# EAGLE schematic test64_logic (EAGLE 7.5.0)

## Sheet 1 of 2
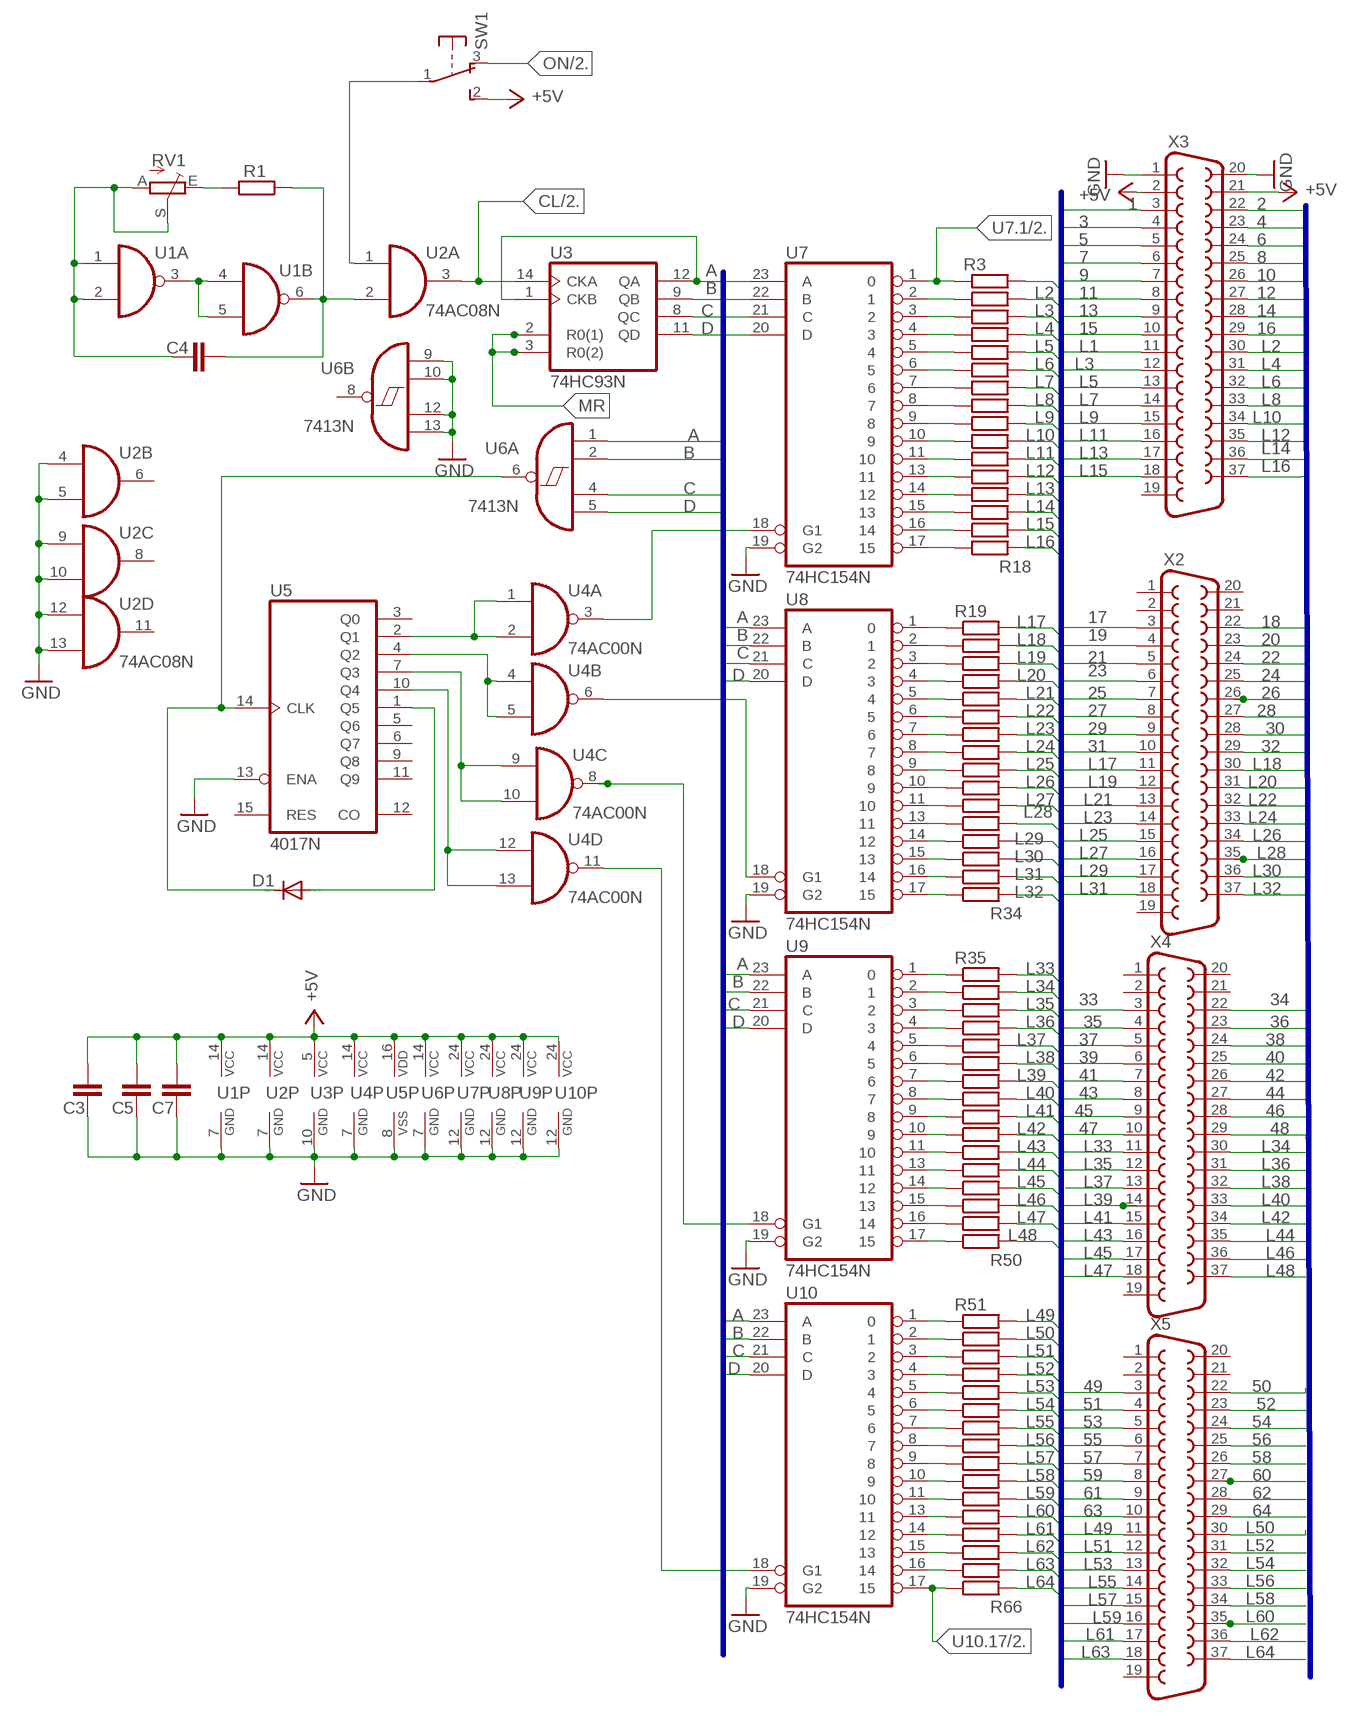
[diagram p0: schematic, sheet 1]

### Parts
C3  C-EUC1206  [C1206]
C4  C-EUC1206  [C1206]
C5  C-EUC1206  [C1206]
C7  C-EUC1206  [C1206]
D1  1N4148DO35-7  [DO35-7]
R1  R-EU_R1206  [R1206]
R3  R-EU_R1206  [R1206]
R4  R-EU_R1206  [R1206]
R5  R-EU_R1206  [R1206]
R6  R-EU_R1206  [R1206]
R7  R-EU_R1206  [R1206]
R8  R-EU_R1206  [R1206]
R9  R-EU_R1206  [R1206]
R10  R-EU_R1206  [R1206]
R11  R-EU_R1206  [R1206]
R12  R-EU_R1206  [R1206]
R13  R-EU_R1206  [R1206]
R14  R-EU_R1206  [R1206]
R15  R-EU_R1206  [R1206]
R16  R-EU_R1206  [R1206]
R17  R-EU_R1206  [R1206]
R18  R-EU_R1206  [R1206]
R19  R-EU_R1206  [R1206]
R20  R-EU_R1206  [R1206]
R21  R-EU_R1206  [R1206]
R22  R-EU_R1206  [R1206]
R23  R-EU_R1206  [R1206]
R24  R-EU_R1206  [R1206]
R25  R-EU_R1206  [R1206]
R26  R-EU_R1206  [R1206]
R27  R-EU_R1206  [R1206]
R28  R-EU_R1206  [R1206]
R29  R-EU_R1206  [R1206]
R30  R-EU_R1206  [R1206]
R31  R-EU_R1206  [R1206]
R32  R-EU_R1206  [R1206]
R33  R-EU_R1206  [R1206]
R34  R-EU_R1206  [R1206]
R35  R-EU_R1206  [R1206]
R36  R-EU_R1206  [R1206]
R37  R-EU_R1206  [R1206]
R38  R-EU_R1206  [R1206]
R39  R-EU_R1206  [R1206]
R40  R-EU_R1206  [R1206]
R41  R-EU_R1206  [R1206]
R42  R-EU_R1206  [R1206]
R43  R-EU_R1206  [R1206]
R44  R-EU_R1206  [R1206]
R45  R-EU_R1206  [R1206]
R46  R-EU_R1206  [R1206]
R47  R-EU_R1206  [R1206]
R48  R-EU_R1206  [R1206]
R49  R-EU_R1206  [R1206]
R50  R-EU_R1206  [R1206]
R51  R-EU_R1206  [R1206]
R52  R-EU_R1206  [R1206]
R53  R-EU_R1206  [R1206]
R54  R-EU_R1206  [R1206]
R55  R-EU_R1206  [R1206]
R56  R-EU_R1206  [R1206]
R57  R-EU_R1206  [R1206]
R58  R-EU_R1206  [R1206]
R59  R-EU_R1206  [R1206]
R60  R-EU_R1206  [R1206]
R61  R-EU_R1206  [R1206]
R62  R-EU_R1206  [R1206]
R63  R-EU_R1206  [R1206]
R64  R-EU_R1206  [R1206]
R65  R-EU_R1206  [R1206]
R66  R-EU_R1206  [R1206]
RV1  TRIM_EU-CT6  [CT6]
SW1  9077-1  [9077-1]
U1  74AC00N  [DIL14]
U2  74AC08N  [DIL14]
U3  74HC93N  [DIL14]
U4  74AC00N  [DIL14]
U5  4017N  [DIL16]
U6  7413N  [DIL14]
U7  74HC154N  [DIL24-6]
U8  74HC154N  [DIL24-6]
U9  74HC154N  [DIL24-6]
U10  74HC154N  [DIL24-6]
X2  F37V  [F37V]
X3  F37V  [F37V]
X4  F37V  [F37V]
X5  F37V  [F37V]

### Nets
1: X3.3 ; also sheet 2
2: X3.22 ; also sheet 2
3: X3.4 ; also sheet 2
4: X3.23 ; also sheet 2
5: X3.5 ; also sheet 2
6: X3.24 ; also sheet 2
7: X3.6 ; also sheet 2
8: X3.25 ; also sheet 2
9: X3.7 ; also sheet 2
10: X3.26 ; also sheet 2
11: X3.8 ; also sheet 2
12: X3.27 ; also sheet 2
13: X3.9 ; also sheet 2
14: X3.28 ; also sheet 2
15: X3.10 ; also sheet 2
16: X3.29 ; also sheet 2
17: X2.3 ; also sheet 2
18: X2.22 ; also sheet 2
19: X2.4 ; also sheet 2
20: X2.23 ; also sheet 2
21: X2.5 ; also sheet 2
22: X2.24 ; also sheet 2
23: X2.6 ; also sheet 2
24: X2.25 ; also sheet 2
25: X2.7 ; also sheet 2
26: X2.26 ; also sheet 2
27: X2.8 ; also sheet 2
28: X2.27 ; also sheet 2
29: X2.9 ; also sheet 2
30: X2.28 ; also sheet 2
31: X2.10 ; also sheet 2
32: X2.29 ; also sheet 2
33: X4.3 ; also sheet 2
34: X4.22 ; also sheet 2
35: X4.4 ; also sheet 2
36: X4.23 ; also sheet 2
37: X4.5 ; also sheet 2
38: X4.24 ; also sheet 2
39: X4.6 ; also sheet 2
40: X4.25 ; also sheet 2
41: X4.7 ; also sheet 2
42: X4.26 ; also sheet 2
43: X4.8 ; also sheet 2
44: X4.27 ; also sheet 2
45: X4.9 ; also sheet 2
46: X4.28 ; also sheet 2
47: X4.10 ; also sheet 2
48: X4.29 ; also sheet 2
49: X5.3 ; also sheet 2
50: X5.22 ; also sheet 2
51: X5.4 ; also sheet 2
52: X5.23 ; also sheet 2
53: X5.5 ; also sheet 2
54: X5.24 ; also sheet 2
55: X5.6 ; also sheet 2
56: X5.25 ; also sheet 2
57: X5.7 ; also sheet 2
58: X5.26 ; also sheet 2
59: X5.8 ; also sheet 2
60: X5.27 ; also sheet 2
61: X5.9 ; also sheet 2
62: X5.28 ; also sheet 2
63: X5.10 ; also sheet 2
64: X5.29 ; also sheet 2
+5V: C3.2 C5.2 C7.2 SW1.2(S) U1.14(P:VCC) U2.14(P:VCC) U3.5(VCC) U4.14(P:VCC) U5.16(VDD) U6.14(P:VCC) U7.24(VCC) U8.24(VCC) U9.24(VCC) U10.24(VCC) X3.2 X3.21 ; also sheet 2
A: U3.1(CKB) U3.12(QA) U6.1(A:I0) U7.23(A) U8.23(A) U9.23(A) U10.23(A)
B: U3.9(QB) U6.2(A:I1) U7.22(B) U8.22(B) U9.22(B) U10.22(B)
C: U3.8(QC) U6.4(A:I2) U7.21(C) U8.21(C) U9.21(C) U10.21(C)
CL: U2.3(A:O) U3.14(CKA) ; also sheet 2
D: U3.11(QD) U6.5(A:I3) U7.20(D) U8.20(D) U9.20(D) U10.20(D)
GND: C3.1 C5.1 C7.1 U1.7(P:GND) U2.4(B:I0) U2.5(B:I1) U2.7(P:GND) U2.9(C:I0) U2.10(C:I1) U2.12(D:I0) U2.13(D:I1) U3.10(GND) U4.7(P:GND) U5.8(VSS) U5.13(ENA) U6.7(P:GND) U6.9(B:I0) U6.10(B:I1) U6.12(B:I2) U6.13(B:I3) U7.12(GND) U7.19(G2) U8.12(GND) U8.19(G2) U9.12(GND) U9.19(G2) U10.12(GND) U10.19(G2) X3.1 X3.20 ; also sheet 2
L1: R3.2 X3.11
L2: R4.2 X3.30
L3: R5.2 X3.12
L4: R6.2 X3.31
L5: R7.2 X3.13
L6: R8.2 X3.32
L7: R9.2 X3.14
L8: R10.2 X3.33
L9: R11.2 X3.15
L10: R12.2 X3.34
L11: R13.2 X3.16
L12: R14.2 X3.35
L13: R15.2 X3.17
L14: R16.2 X3.36
L15: R17.2 X3.18
L16: R18.2 X3.37
L17: R19.2 X2.11
L18: R20.2 X2.30
L19: R21.2 X2.12
L20: R22.2 X2.31
L21: R23.2 X2.13
L22: R24.2 X2.32
L23: R25.2 X2.14
L24: R26.2 X2.33
L25: R27.2 X2.15
L26: R28.2 X2.34
L27: R29.2 X2.16
L28: R30.2 X2.35
L29: R31.2 X2.17
L30: R32.2 X2.36
L31: R33.2 X2.18
L32: R34.2 X2.37
L33: R35.2 X4.11
L34: R36.2 X4.30
L35: R37.2 X4.12
L36: R38.2 X4.31
L37: R39.2 X4.13
L38: R40.2 X4.32
L39: R41.2 X4.14
L40: R42.2 X4.33
L41: R43.2 X4.15
L42: R44.2 X4.34
L43: R45.2 X4.16
L44: R46.2 X4.35
L45: R47.2 X4.17
L46: R48.2 X4.36
L47: R49.2 X4.18
L48: R50.2 X4.37
L49: R51.2 X5.11
L50: R52.2 X5.30
L51: R53.2 X5.12
L52: R54.2 X5.31
L53: R55.2 X5.13
L54: R56.2 X5.32
L55: R57.2 X5.14
L56: R58.2 X5.33
L57: R59.2 X5.15
L58: R60.2 X5.34
L59: R61.2 X5.16
L60: R62.2 X5.35
L61: R63.2 X5.17
L62: R64.2 X5.36
L63: R65.2 X5.18
L64: R66.2 X5.37
MR: U3.2(R0(1)) U3.3(R0(2))
N$1: U1.3(A:O) U1.4(B:I0) U1.5(B:I1)
N$2: C4.1 RV1.A RV1.S U1.1(A:I0) U1.2(A:I1)
N$3: C4.2 R1.1 U1.6(B:O) U2.2(A:I1)
N$5: R1.2 RV1.E
N$7: R4.1 U7.2
N$8: R5.1 U7.3
N$9: R6.1 U7.4
N$10: R7.1 U7.5
N$11: R8.1 U7.6
N$12: R9.1 U7.7
N$13: R10.1 U7.8
N$14: R11.1 U7.9
N$15: R12.1 U7.10
N$16: R13.1 U7.11
N$17: R14.1 U7.13
N$18: R15.1 U7.14
N$19: R16.1 U7.15
N$20: R17.1 U7.16
N$21: R18.1 U7.17
N$22: R19.1 U8.1
N$23: R20.1 U8.2
N$24: R21.1 U8.3
N$25: R22.1 U8.4
N$26: R23.1 U8.5
N$27: R24.1 U8.6
N$28: R25.1 U8.7
N$29: R26.1 U8.8
N$30: R27.1 U8.9
N$31: R28.1 U8.10
N$32: R29.1 U8.11
N$33: R30.1 U8.13
N$34: R31.1 U8.14
N$35: R32.1 U8.15
N$36: R33.1 U8.16
N$37: R34.1 U8.17
N$38: R35.1 U9.1
N$39: R36.1 U9.2
N$40: R37.1 U9.3
N$41: R38.1 U9.4
N$42: R39.1 U9.5
N$43: R40.1 U9.6
N$44: R41.1 U9.7
N$45: R42.1 U9.8
N$46: R43.1 U9.9
N$47: R44.1 U9.10
N$48: R45.1 U9.11
N$49: R46.1 U9.13
N$50: R47.1 U9.14
N$51: R48.1 U9.15
N$52: R49.1 U9.16
N$53: R50.1 U9.17
N$54: R51.1 U10.1
N$55: R52.1 U10.2
N$56: R53.1 U10.3
N$57: R54.1 U10.4
N$58: R55.1 U10.5
N$59: R56.1 U10.6
N$60: R57.1 U10.7
N$61: R58.1 U10.8
N$62: R59.1 U10.9
N$63: R60.1 U10.10
N$64: R61.1 U10.11
N$65: R62.1 U10.13
N$66: R63.1 U10.14
N$67: R64.1 U10.15
N$68: R65.1 U10.16
N$70: U4.1(A:I0) U4.2(A:I1) U5.2(Q1)
N$71: U4.4(B:I0) U4.5(B:I1) U5.4(Q2)
N$72: U4.9(C:I0) U4.10(C:I1) U5.7(Q3)
N$73: D1.A U5.1(Q5)
N$74: U4.3(A:O) U7.18(G1)
N$75: U4.6(B:O) U8.18(G1)
N$76: U4.8(C:O) U9.18(G1)
N$77: U4.11(D:O) U10.18(G1)
N$78: D1.C U5.14(CLK) U6.6(A:O)
N$79: U4.12(D:I0) U4.13(D:I1) U5.10(Q4)
N$80: SW1.1(P) U2.1(A:I0)
ON: SW1.3(O) ; also sheet 2
U7.1: R3.1 U7.1 ; also sheet 2
U10.17: R66.1 U10.17 ; also sheet 2
Unconnected: U1.8(C:O) U1.9(C:I0) U1.10(C:I1) U1.11(D:O) U1.12(D:I0) U1.13(D:I1) U2.6(B:O) U2.8(C:O) U2.11(D:O) U5.3(Q0) U5.5(Q6) U5.6(Q7) U5.9(Q8) U5.11(Q9) U5.12(CO) U5.15(RES) U6.8(B:O) X2.1 X2.2 X2.19 X2.20 X2.21 X3.19 X4.1 X4.2 X4.19 X4.20 X4.21 X5.1 X5.2 X5.19 X5.20 X5.21

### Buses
B$1
B$2

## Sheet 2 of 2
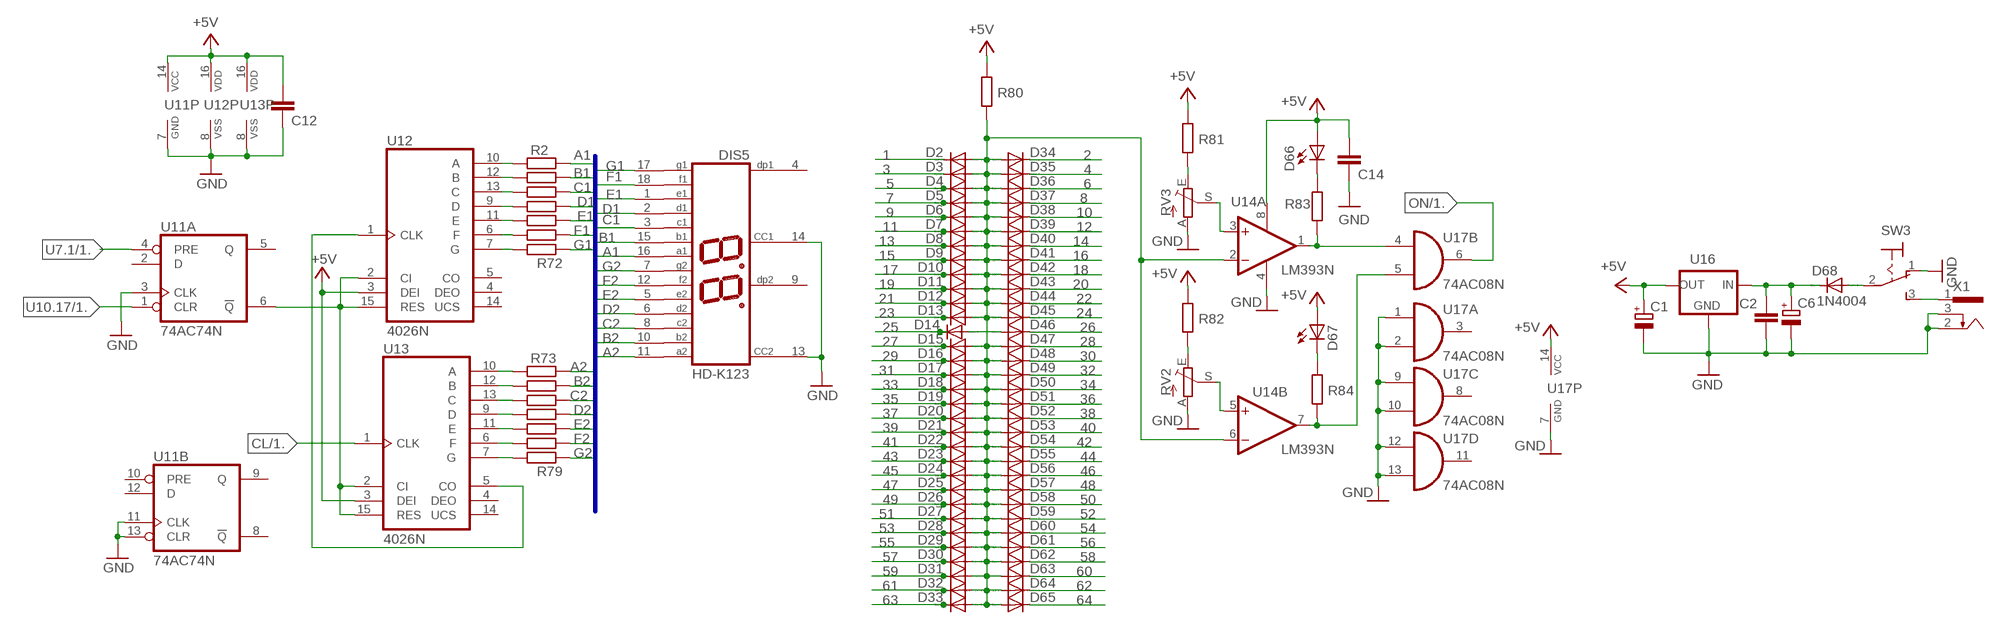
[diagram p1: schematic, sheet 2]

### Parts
C1  CPOL-EUC/6032-28W  [C/6032-28W]
C2  C-EUC1206  [C1206]
C6  CPOL-EUC/6032-28W  [C/6032-28W]
C12  C-EUC1206  [C1206]
C14  C-EUC1206  [C1206]
D2  1N4148DO35-7  [DO35-7]
D3  1N4148DO35-7  [DO35-7]
D4  1N4148DO35-7  [DO35-7]
D5  1N4148DO35-7  [DO35-7]
D6  1N4148DO35-7  [DO35-7]
D7  1N4148DO35-7  [DO35-7]
D8  1N4148DO35-7  [DO35-7]
D9  1N4148DO35-7  [DO35-7]
D10  1N4148DO35-7  [DO35-7]
D11  1N4148DO35-7  [DO35-7]
D12  1N4148DO35-7  [DO35-7]
D13  1N4148DO35-7  [DO35-7]
D14  1N4148DO35-7  [DO35-7]
D15  1N4148DO35-7  [DO35-7]
D16  1N4148DO35-7  [DO35-7]
D17  1N4148DO35-7  [DO35-7]
D18  1N4148DO35-7  [DO35-7]
D19  1N4148DO35-7  [DO35-7]
D20  1N4148DO35-7  [DO35-7]
D21  1N4148DO35-7  [DO35-7]
D22  1N4148DO35-7  [DO35-7]
D23  1N4148DO35-7  [DO35-7]
D24  1N4148DO35-7  [DO35-7]
D25  1N4148DO35-7  [DO35-7]
D26  1N4148DO35-7  [DO35-7]
D27  1N4148DO35-7  [DO35-7]
D28  1N4148DO35-7  [DO35-7]
D29  1N4148DO35-7  [DO35-7]
D30  1N4148DO35-7  [DO35-7]
D31  1N4148DO35-7  [DO35-7]
D32  1N4148DO35-7  [DO35-7]
D33  1N4148DO35-7  [DO35-7]
D34  1N4148DO35-7  [DO35-7]
D35  1N4148DO35-7  [DO35-7]
D36  1N4148DO35-7  [DO35-7]
D37  1N4148DO35-7  [DO35-7]
D38  1N4148DO35-7  [DO35-7]
D39  1N4148DO35-7  [DO35-7]
D40  1N4148DO35-7  [DO35-7]
D41  1N4148DO35-7  [DO35-7]
D42  1N4148DO35-7  [DO35-7]
D43  1N4148DO35-7  [DO35-7]
D44  1N4148DO35-7  [DO35-7]
D45  1N4148DO35-7  [DO35-7]
D46  1N4148DO35-7  [DO35-7]
D47  1N4148DO35-7  [DO35-7]
D48  1N4148DO35-7  [DO35-7]
D49  1N4148DO35-7  [DO35-7]
D50  1N4148DO35-7  [DO35-7]
D51  1N4148DO35-7  [DO35-7]
D52  1N4148DO35-7  [DO35-7]
D53  1N4148DO35-7  [DO35-7]
D54  1N4148DO35-7  [DO35-7]
D55  1N4148DO35-7  [DO35-7]
D56  1N4148DO35-7  [DO35-7]
D57  1N4148DO35-7  [DO35-7]
D58  1N4148DO35-7  [DO35-7]
D59  1N4148DO35-7  [DO35-7]
D60  1N4148DO35-7  [DO35-7]
D61  1N4148DO35-7  [DO35-7]
D62  1N4148DO35-7  [DO35-7]
D63  1N4148DO35-7  [DO35-7]
D64  1N4148DO35-7  [DO35-7]
D65  1N4148DO35-7  [DO35-7]
D66  LED5MM  [LED5MM]
D67  LED5MM  [LED5MM]
D68  1N4004  [DO41-10]
DIS5  HD-K123  [HDSP-R]
R2  R-EU_R1206  [R1206]
R67  R-EU_R1206  [R1206]
R68  R-EU_R1206  [R1206]
R69  R-EU_R1206  [R1206]
R70  R-EU_R1206  [R1206]
R71  R-EU_R1206  [R1206]
R72  R-EU_R1206  [R1206]
R73  R-EU_R1206  [R1206]
R74  R-EU_R1206  [R1206]
R75  R-EU_R1206  [R1206]
R76  R-EU_R1206  [R1206]
R77  R-EU_R1206  [R1206]
R78  R-EU_R1206  [R1206]
R79  R-EU_R1206  [R1206]
R80  R-EU_R1206  [R1206]
R81  R-EU_R1206  [R1206]
R82  R-EU_R1206  [R1206]
R83  R-EU_R1206  [R1206]
R84  R-EU_R1206  [R1206]
RV2  TRIM_EU-CT6  [CT6]
RV3  TRIM_EU-CT6  [CT6]
SW3  320-916  [320-916]
U11  74AC74N  [DIL14]
U12  4026N  [DIL16]
U13  4026N  [DIL16]
U14  LM393N  [DIL08]
U16  78XXL  [78XXL]
U17  74AC08N  [DIL14]
X1  733980-62  [733980-62]

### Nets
1: D2.C ; also sheet 1
2: D34.C ; also sheet 1
3: D3.C ; also sheet 1
4: D35.C ; also sheet 1
5: D4.C ; also sheet 1
6: D36.C ; also sheet 1
7: D5.C ; also sheet 1
8: D37.C ; also sheet 1
9: D6.C ; also sheet 1
10: D38.C ; also sheet 1
11: D7.C ; also sheet 1
12: D39.C ; also sheet 1
13: D8.C ; also sheet 1
14: D40.C ; also sheet 1
15: D9.C ; also sheet 1
16: D41.C ; also sheet 1
17: D10.C ; also sheet 1
18: D42.C ; also sheet 1
19: D11.C ; also sheet 1
20: D43.C ; also sheet 1
21: D12.C ; also sheet 1
22: D44.C ; also sheet 1
23: D13.C ; also sheet 1
24: D45.C ; also sheet 1
25: D14.C ; also sheet 1
26: D46.C ; also sheet 1
27: D15.C ; also sheet 1
28: D47.C ; also sheet 1
29: D16.C ; also sheet 1
30: D48.C ; also sheet 1
31: D17.C ; also sheet 1
32: D49.C ; also sheet 1
33: D18.C ; also sheet 1
34: D50.C ; also sheet 1
35: D19.C ; also sheet 1
36: D51.C ; also sheet 1
37: D20.C ; also sheet 1
38: D52.C ; also sheet 1
39: D21.C ; also sheet 1
40: D53.C ; also sheet 1
41: D22.C ; also sheet 1
42: D54.C ; also sheet 1
43: D23.C ; also sheet 1
44: D55.C ; also sheet 1
45: D24.C ; also sheet 1
46: D56.C ; also sheet 1
47: D25.C ; also sheet 1
48: D57.C ; also sheet 1
49: D26.C ; also sheet 1
50: D58.C ; also sheet 1
51: D27.C ; also sheet 1
52: D59.C ; also sheet 1
53: D28.C ; also sheet 1
54: D60.C ; also sheet 1
55: D29.C ; also sheet 1
56: D61.C ; also sheet 1
57: D30.C ; also sheet 1
58: D62.C ; also sheet 1
59: D31.C ; also sheet 1
60: D63.C ; also sheet 1
61: D32.C ; also sheet 1
62: D64.C ; also sheet 1
63: D33.C ; also sheet 1
64: D65.C ; also sheet 1
+5V: C1.+ C12.2 C14.2 D66.A D67.A R80.1 R81.1 R82.1 U11.14(P:VCC) U12.3(DEI) U12.16(VDD) U13.3(DEI) U13.16(VDD) U14.8(P:V+) U16.OUT U17.14(P:VCC) ; also sheet 1
A1: DIS5.16(A1) R2.1
A2: DIS5.11(A2) R73.1
B1: DIS5.15(B1) R67.1
B2: DIS5.10(B2) R74.1
C1: DIS5.3(C1) R68.1
C2: DIS5.8(C2) R75.1
CL: U13.1(CLK) ; also sheet 1
D1: DIS5.2(D1) R69.1
D2: DIS5.6(D2) R76.1
E1: DIS5.1(E1) R70.1
E2: DIS5.5(E2) R77.1
F1: DIS5.18(F1) R71.1
F2: DIS5.12(F2) R78.1
G1: DIS5.17(G1) R72.1
G2: DIS5.7(G2) R79.1
GND: C1.- C2.2 C6.- C12.1 C14.1 DIS5.13(CC2) DIS5.14(CC1) RV2.A RV3.A SW3.1(O) U11.3(A:CLK) U11.7(P:GND) U11.11(B:CLK) U11.13(B:CLR) U12.8(VSS) U13.8(VSS) U14.4(P:V-) U16.GND U17.1(A:I0) U17.2(A:I1) U17.7(P:GND) U17.9(C:I0) U17.10(C:I1) U17.12(D:I0) U17.13(D:I1) X1.2 X1.3 ; also sheet 1
N$6: U11.6(A:!Q) U12.2(CI) U12.15(RES) U13.2(CI) U13.15(RES)
N$69: U12.1(CLK) U13.5(CO)
N$81: R2.2 U12.10(A)
N$82: R67.2 U12.12(B)
N$83: R68.2 U12.13(C)
N$84: R69.2 U12.9(D)
N$85: R70.2 U12.11(E)
N$86: R71.2 U12.6(F)
N$87: R72.2 U12.7(G)
N$88: R73.2 U13.10(A)
N$89: R74.2 U13.12(B)
N$90: R75.2 U13.13(C)
N$91: R76.2 U13.9(D)
N$92: R77.2 U13.11(E)
N$93: R78.2 U13.6(F)
N$94: R79.2 U13.7(G)
N$95: D68.A SW3.2(P)
N$109: D2.A D3.A D4.A D5.A D6.A D7.A D8.A D9.A D10.A D11.A D12.A D13.A D14.A D15.A D16.A D17.A D18.A D19.A D20.A D21.A D22.A D23.A D24.A D25.A D26.A D27.A D28.A D29.A D30.A D31.A D32.A D33.A D34.A D35.A D36.A D37.A D38.A D39.A D40.A D41.A D42.A D43.A D44.A D45.A D46.A D47.A D48.A D49.A D50.A D51.A D52.A D53.A D54.A D55.A D56.A D57.A D58.A D59.A D60.A D61.A D62.A D63.A D64.A D65.A R80.2 U14.2(A:-IN) U14.6(B:-IN)
N$110: R81.2 RV3.E
N$111: R82.2 RV2.E
N$112: RV2.S U14.5(B:+IN)
N$113: RV3.S U14.3(A:+IN)
N$114: D66.K(C) R83.1
N$115: D67.K(C) R84.1
N$116: R84.2 U14.7(B:OUT) U17.5(B:I1)
N$117: R83.2 U14.1(A:OUT) U17.4(B:I0)
N$118: C2.1 C6.+ D68.C U16.IN
N$119: SW3.3(S) X1.1
ON: U17.6(B:O) ; also sheet 1
U7.1: U11.4(A:PRE) ; also sheet 1
U10.17: U11.1(A:CLR) ; also sheet 1
Unconnected: DIS5.4(DP1) DIS5.9(DP2) U11.2(A:D) U11.5(A:Q) U11.8(B:!Q) U11.9(B:Q) U11.10(B:PRE) U11.12(B:D) U12.4(DEO) U12.5(CO) U12.14(UCS) U13.4(DEO) U13.14(UCS) U17.3(A:O) U17.8(C:O) U17.11(D:O)

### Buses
B$3

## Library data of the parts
C1 C6 = rcl:CPOL-EU: POLARIZED CAPACITOR, European symbol
C2-C5 C7 C12 C14 = rcl:C-EU: CAPACITOR, European symbol
D1-D65 = diode:1N4148: DIODE
D66 D67 = led:LED: LED
D68 = diode:1N4004: DIODE
DIS5 = display-hp:HD-K123: LED DISPLAY 2 x 1 character 7 segment, decimal points right; OC_FARNELL: unknown; OC_NEWARK: unknown
R1-R84 = rcl:R-EU_: RESISTOR, European symbol
RV1-RV3 = pot:TRIM_EU-: POTENTIOMETER
SW1 = switch-misc:9077-1: MARQUARDT SWITCH 9077.0100 Distributor: Buerklin
SW3 = switch:320-916: TOGGLE SWITCH distributor RS Components
U1 U4 = 74xx-eu:74*00: Quad 2-input NAND gate
U2 U17 = 74xx-eu:74*08: Quad 2-input AND gate
U3 = 74xx-eu:74*93: Decade, divide by twelve and binary COUNTER
U5 = 40xx:4017: COUNTER/DIVIDER
U6 = 74xx-eu:74*13: Dual 4-input NAND schmitt trigger
U7-U10 = 74xx-eu:74*154: 4-line to 16-line data SELECTOR/MULTIPLEXER
U11 = 74xx-eu:74*74: Dual D type positive edge triggered FLIP FLOP, preset and clear
U12 U13 = 40xx:4026: Decade COUNTER/DIVIDER, 7-seg. outputs
U14 = linear:LM393: COMPARATOR
U16 = v-reg:78XXL: VOLTAGE REGULATOR
X1 = con-conrad:73398?: FEMALE PRINT CONNECTOR Niedervolt-Steckverbinder Distributor Conrad
X2-X5 = con-subd:F37: SUB-D; OC_FARNELL: unknown; OC_NEWARK: unknown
